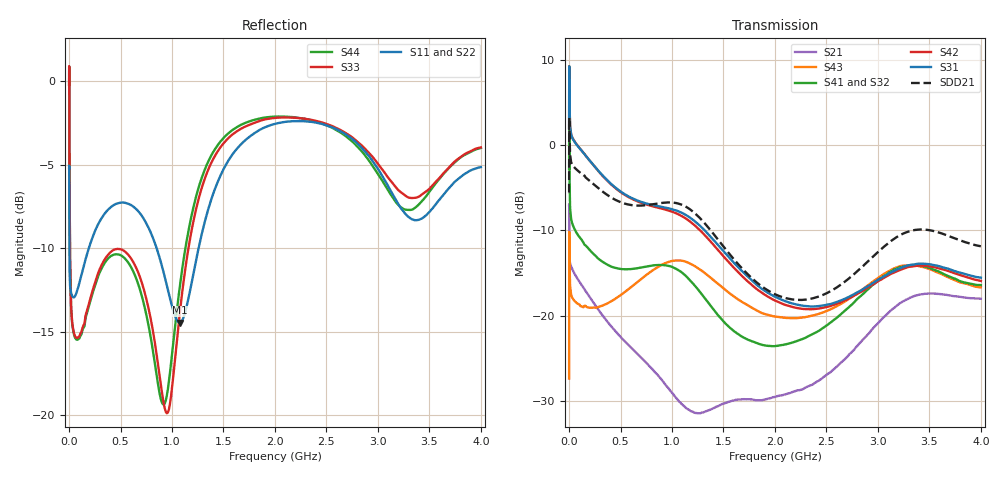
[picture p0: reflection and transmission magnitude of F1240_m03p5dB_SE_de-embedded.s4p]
! Integrated Device Technology
! Corporate Headquarters
! 6024 Silver Creek Valley Road
! San Jose, CA 95138  USA
! Phone:  1-408-284-8200
! Toll Free:  1-800-223-1366
! Webpage:  http://www.idt.com/
! Timing and RF Division
! 515 Groton Road, Suite 102
! Westford, MA 01886-6024
! Device:  F1240
! Description: Dual Intermediate Frequency Digital Variable Gain Amplifier
! Frequency:  10.0 -  500.00 MHz
! Package:  5x5 mm QFN Plastic Package: 32 pin
! Ports:  8 RF, 20 DC
!  Pin  1  = GA3 / Data  Pin 17  = RF OUT_B+
!  Pin  2  = GA4 / CLK  Pin 18  = RF OUT_B-
!  Pin  3  = GA5  Pin 19  = STBY_B
!  Pin  4  = VMODE  Pin 20  = Ground
!  Pin  5  = No Connect  Pin 21  = Ground
!  Pin  6  = GB5  Pin 22  = STB_A
!  Pin  7  = GB4  Pin 23  = RF OUT_A-  = Port 4
!  Pin  8  = GB3  Pin 24  = RF OUT_A+  = Port 3
!  Pin  9  = GB2  Pin 25  = GA0
!  Pin 10  = GB1  Pin 26  = ISET_A
!  Pin 11  = RF IN_B+  Pin 27  = VCC
!  Pin 12  = RF IN_B-  Pin 28  = Ground
!  Pin 13  = Ground  Pin 29  = RF IN_A-  = Port 2
!  Pin 14  = VCC  Pin 30  = RF IN_A+  = Port 1
!  Pin 15  = ISET_B  Pin 31  = GA1
!  Pin 16  = GB0  Pin 32  = GA2 / CSb
! Gain  = +19.5 dB
! State  = 1
! Voltage  = +5.00 V
! Current  = 85.292 mA (one channel only)
! Temperture  =  +25 C
! Test Date  =  2017-10-18
! Board  =  EB4031
! Data:  The device was measured on a custom evaluation board which has
!  individual transmission lines to the RF pins.  Data was collected
!  using a calibrated network analyzer.  The evaluation board was
!  de-embedded using Automatic Fixture Removal.
!  The reference plane is the edge of the package pin.
!  Only Channel A was measured.
!  This data is in single-ended operation.  If your needs are balanced
!  or differential S-parameters then this file needs to be used a
!  linear simulator.
! File Date:  2017-11-10  MJV
! Note:
!  Integrated Device Technology supplies this data as a sample of measured
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# Hz S dB R 100
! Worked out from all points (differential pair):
!   410 points, 500 kHz to 4 GHz, reference 100 ohm
!   strongest paths, dB at 500 kHz, 930 MHz, 1.96 GHz, 2.98 GHz, 4 GHz:
!     S31: 2.0, -7.3, -17.5, -16.0, -15.5
!     S42: 2.0, -7.5, -18.0, -16.1, -15.9
!     S41: -2.8, -14.1, -23.6, -16.1, -16.4
!     S32: -2.7, -14.3, -23.5, -16.5, -16.9
!     S43: -27.4, -13.9, -20.0, -15.8, -16.7
!     S21: -7.0, -28.0, -29.7, -21.1, -18.0
!   taken as a pair (ports 1,2 in; 3,4 out), SDD21 dB: -5.6, -6.7, -17.2, -12.8, -11.9
!   lowest |S11| = -14.5 dB at 1.08 GHz (marker M1), VSWR 1.47, Z = 69.7 - j10.9 ohm
!   |S11| at or under -10 dB: 3.251 MHz to 191.6 MHz (188.4 MHz wide, 193 % of centre); 850.4 MHz to 1.258 GHz (407.7 MHz wide, 38.7 % of centre)
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500000  -5.20 -5.5  -7.03 -5.9  -30.86 79.3  -35.46 77.6
        -7.04 -5.9  -5.20 -5.5  -35.44 76.3  -30.85 80.4
        1.96 -109.1  -2.75 -111.5  -0.20 0.4  -27.35 -40.8
        -2.78 -110.4  1.96 -107.9  -27.37 -40.9  -0.21 2.7
2000000  -7.47 -32.4  -9.85 -33.4  -21.92 25.7  -27.36 6.6
         -9.85 -33.4  -7.44 -32.5  -27.31 6.3  -21.90 26.0
         8.82 -179.1  3.36 162.2  -0.12 -51.8  -10.18 -142.3
         3.32 162.5  8.83 -178.8  -10.17 -142.3  -0.16 -51.4
4000000  -10.79 -28.7  -13.06 -23.3  -22.43 7.1  -30.50 -13.1
         -13.07 -23.3  -10.79 -29.0  -30.46 -13.3  -22.42 7.2
         5.52 158.7  -2.58 138.1  -4.63 -85.3  -12.84 174.0
         -2.62 138.3  5.53 158.9  -12.84 174.0  -4.67 -85.3
4e8  -7.57 -140.5  -21.12 -104.8  -26.46 -83.8  -36.09 -65.5
     -21.12 -104.7  -7.47 -141.7  -36.22 -64.1  -26.61 -84.2
     -4.46 55.7  -14.27 4.7  -10.25 -163.8  -18.46 40.0
     -14.20 3.9  -4.52 54.4  -18.38 39.5  -10.50 -164.4
1.08e9  -14.45 -156.5  -30.58 160.8  -25.34 143.0  -32.60 -177.8
        -30.16 159.6  -14.49 -154.4  -32.58 -173.2  -26.18 142.7
        -7.85 -103.2  -15.01 162.5  -13.63 -106.7  -13.72 -141.5
        -14.80 157.8  -8.22 -105.6  -13.53 -141.6  -12.10 -106.8
2.86e9  -4.11 101.9  -22.78 -26.3  -26.40 -152.7  -28.65 -136.9
        -22.75 -26.4  -3.87 102.7  -29.41 -124.6  -27.66 -146.9
        -16.86 -66.5  -17.77 -151.1  -3.95 102.1  -17.68 -81.8
        -17.42 -162.0  -17.04 -63.4  -16.83 -79.6  -4.32 95.2
4e9  -5.14 -134.8  -18.03 110.6  -25.09 -38.8  -26.12 -23.1
     -18.01 110.4  -4.81 -133.4  -26.90 -7.9  -26.90 -31.3
     -15.55 42.2  -16.88 -59.0  -3.96 -133.7  -18.14 64.7
     -16.41 -72.7  -15.93 48.1  -16.69 56.8  -4.00 -143.4
